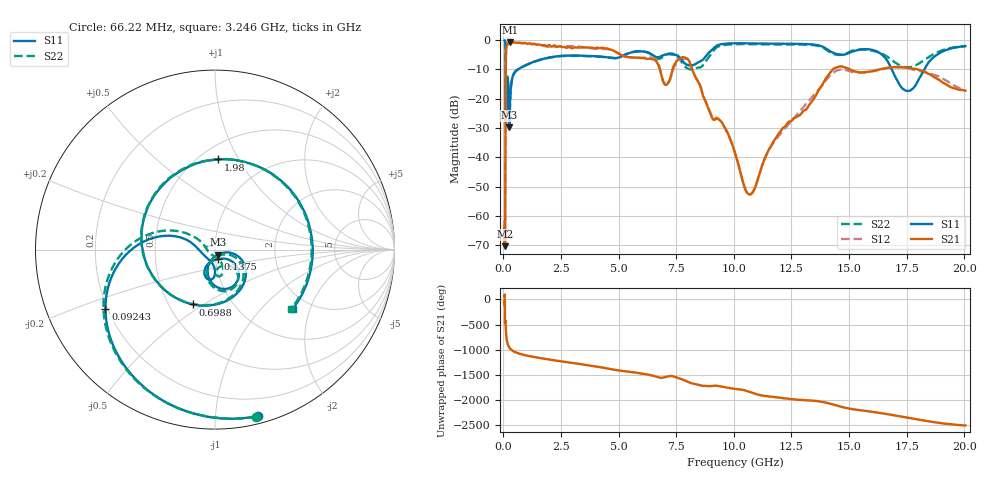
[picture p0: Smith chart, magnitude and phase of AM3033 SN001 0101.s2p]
# Hz S DB R 50
!freq MagS11 AngS11 MagS21 AngS21 MagS12 AngS12 MagS22 AngS22
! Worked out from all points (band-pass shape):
!   1601 points, 50 MHz to 20.05 GHz, reference 50 ohm
!   highest |S21| = -0.70 dB at 301.9 MHz (marker M1); lowest = -70.2 dB at 71.37 MHz (marker M2)
!   |S21| within 3 dB of the highest: 114.7 MHz to 4.789 GHz (4.674 GHz wide, 191 % of centre)
!   lowest |S11| = -29.8 dB at 254.1 MHz (marker M3), VSWR 1.07, Z = 51.5 - j2.95 ohm
!   |S11| at or under -10 dB: 98.91 MHz to 627.2 MHz (528.3 MHz wide, 146 % of centre); 16.85 GHz to 18.27 GHz (1.413 GHz wide, 8.05 % of centre)
!   |S22| runs from -29.4 to -0.1 dB; largest |S21 - S12| = 0.063
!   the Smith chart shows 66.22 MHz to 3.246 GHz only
!   S11 on the Smith chart (normalised r, x): 66.22 MHz: 0.06, -1.29; 92.43 MHz: 0.19, -0.24; 137.5 MHz: 1.03, -0.11; 698.8 MHz: 0.66, -0.45; 1.98 GHz: 0.61, +0.82; 3.246 GHz: 1.63, -1.53
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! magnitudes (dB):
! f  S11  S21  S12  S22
! 50 MHz  -0.2  -61.8  -63.0  -0.1
! 66.22 MHz  -0.4  -67.6  -68.3  -0.4
! 71.37 MHz  -0.5  -70.2  -66.0  -0.5
! 92.43 MHz  -3.2  -23.4  -23.4  -3.2
! 107 MHz  -23.3  -5.4  -5.4  -29.3
! 135.9 MHz  -24.9  -2.1  -2.1  -20.1
! 137.5 MHz  -25.1  -2.1  -2.1  -20.0
! 181.4 MHz  -13.0  -1.4  -1.4  -12.6
! 254.1 MHz  -29.8  -0.8  -0.8  -27.9
! 301.9 MHz  -18.2  -0.7  -0.7  -18.5
! 369.6 MHz  -13.4  -0.8  -0.7  -13.5
! 698.8 MHz  -9.6  -0.9  -1.0  -9.7
! 1.005 GHz  -8.5  -1.3  -1.1  -8.4
! 1.98 GHz  -6.0  -1.7  -2.3  -6.0
! 2.722 GHz  -5.3  -2.6  -2.2  -5.4
! 3.246 GHz  -5.3  -2.6  -2.1  -5.4
! 7.402 GHz  -4.9  -8.6  -9.3  -4.8
! 8.129 GHz  -8.6  -8.6  -8.7  -10.1
! 10.69 GHz  -1.1  -52.6  -52.7  -1.4
! 14.47 GHz  -4.8  -9.3  -10.4  -5.0
! 17.59 GHz  -17.3  -9.5  -9.7  -9.3
! 20.05 GHz  -2.0  -17.3  -17.2  -2.1
